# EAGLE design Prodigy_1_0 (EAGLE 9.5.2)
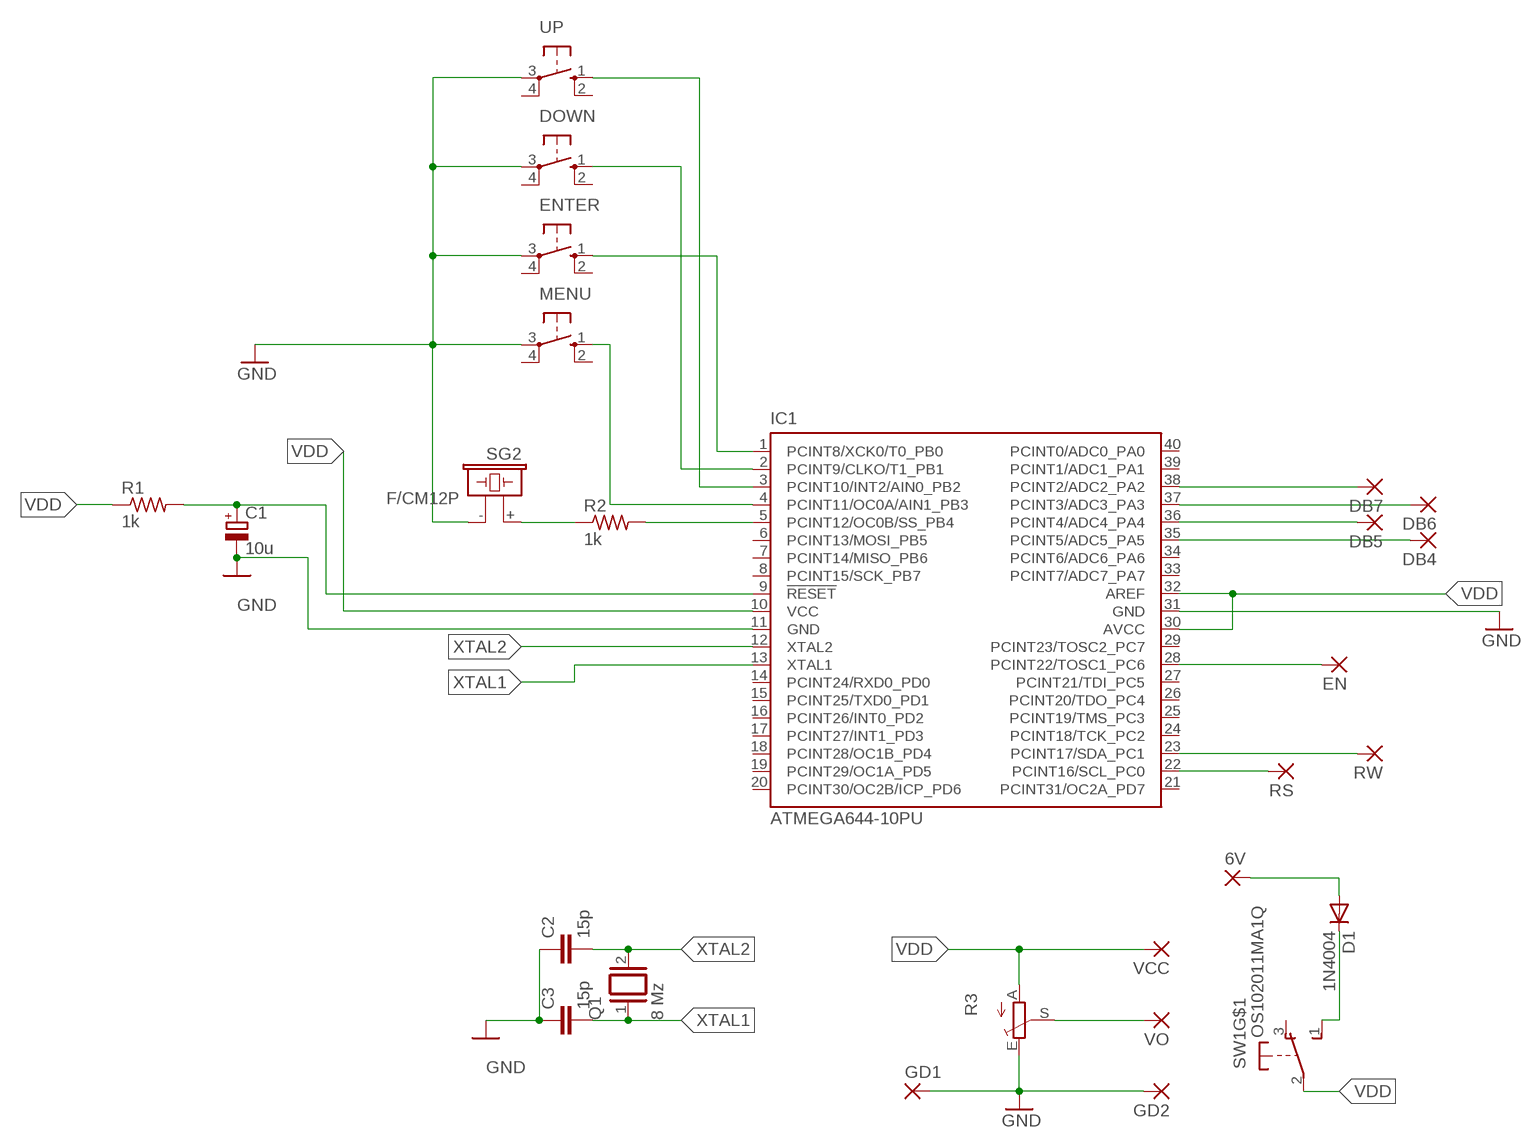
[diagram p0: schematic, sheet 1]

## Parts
6V  3,17/1,1  [3,17/1,1]
C1  10u  CPOL-EUB45181B  [B45181B]
C2  15p  C5/5  [C5B5]
C3  15p  C5/5  [C5B5]
D1  1N4004  [DO41-10]
DB4  3,17/1,1  [3,17/1,1]
DB5  3,17/1,1  [3,17/1,1]
DB6  3,17/1,1  [3,17/1,1]
DB7  3,17/1,1  [3,17/1,1]
DOWN  10-XX  [B3F-10XX]
EN  3,17/1,1  [3,17/1,1]
ENTER  10-XX  [B3F-10XX]
GD1  3,17/1,1  [3,17/1,1]
GD2  3,17/1,1  [3,17/1,1]
IC1  ATMEGA644-10PU  [DIL40]
MENU  10-XX  [B3F-10XX]
Q1  8 Mz  XTAL/S  [QS]
R1  1k  R-US_0204/7  [0204/7]
R2  1k  R-US_0204/7  [0204/7]
R3  TRIM_EU-LI10  [LI10]
RS  3,17/1,1  [3,17/1,1]
RW  3,17/1,1  [3,17/1,1]
SG2  F/CM12P  [F/CM12P]
SW1  OS102011MA1Q  [OS102011MA1Q]
UP  10-XX  [B3F-10XX]
VCC  3,17/1,1  [3,17/1,1]
VO  3,17/1,1  [3,17/1,1]

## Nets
GND: C1.- C2.1 C3.1 DOWN.3(P) ENTER.3(P) GD1.1(P) GD2.1(P) IC1.11(GND) IC1.31(GND) MENU.3(P) R3.E SG2.- UP.3(P)
N$1: ENTER.1(S) IC1.1(PCINT8/XCK0/T0_PB0)
N$2: DOWN.1(S) IC1.2(PCINT9/CLKO/T1_PB1)
N$3: DB7.1(P) IC1.38(PCINT2/ADC2_PA2)
N$4: C1.+ IC1.9(!RESET) R1.2
N$5: IC1.3(PCINT10/INT2/AIN0_PB2) UP.1(S)
N$6: IC1.4(PCINT11/OC0A/AIN1_PB3) MENU.1(S)
N$7: R2.1 SG2.+
N$8: EN.1(P) IC1.28(PCINT22/TOSC1_PC6)
N$9: DB5.1(P) IC1.36(PCINT4/ADC4_PA4)
N$10: IC1.23(PCINT17/SDA_PC1) RW.1(P)
N$11: DB4.1(P) IC1.35(PCINT5/ADC5_PA5)
N$12: DB6.1(P) IC1.37(PCINT3/ADC3_PA3)
N$13: IC1.22(PCINT16/SCL_PC0) RS.1(P)
N$14: D1.C SW1.1(S)
N$15: R3.S VO.1(P)
N$16: 6V.1(P) D1.A
N$17: IC1.5(PCINT12/OC0B/SS_PB4) R2.2
VDD: IC1.10(VCC) IC1.30(AVCC) IC1.32(AREF) R1.1 R3.A SW1.2(P) VCC.1(P)
XTAL1: C3.2 IC1.13(XTAL1) Q1.1
XTAL2: C2.2 IC1.12(XTAL2) Q1.2
Unconnected: DOWN.2(S1) DOWN.4(P1) ENTER.2(S1) ENTER.4(P1) IC1.6(PCINT13/MOSI_PB5) IC1.7(PCINT14/MISO_PB6) IC1.8(PCINT15/SCK_PB7) IC1.14(PCINT24/RXD0_PD0) IC1.15(PCINT25/TXD0_PD1) IC1.16(PCINT26/INT0_PD2) IC1.17(PCINT27/INT1_PD3) IC1.18(PCINT28/OC1B_PD4) IC1.19(PCINT29/OC1A_PD5) IC1.20(PCINT30/OC2B/ICP_PD6) IC1.21(PCINT31/OC2A_PD7) IC1.24(PCINT18/TCK_PC2) IC1.25(PCINT19/TMS_PC3) IC1.26(PCINT20/TDO_PC4) IC1.27(PCINT21/TDI_PC5) IC1.29(PCINT23/TOSC2_PC7) IC1.33(PCINT7/ADC7_PA7) IC1.34(PCINT6/ADC6_PA6) IC1.39(PCINT1/ADC1_PA1) IC1.40(PCINT0/ADC0_PA0) MENU.2(S1) MENU.4(P1) SW1.3(O) SW1.MT1(MT) SW1.MT2(MT) UP.2(S1) UP.4(P1)

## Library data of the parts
6V DB4-DB7 EN GD1 GD2 RS RW VCC VO = wirepad:3,17/1,1: THROUGH-HOLE PAD; OC_NEWARK: unknown
C1 = rcl:CPOL-EU: POLARIZED CAPACITOR, European symbol; SPICEPREFIX: C
C2 C3 = capacitor-wima:C: CAPACITOR; OC_NEWARK: unknown
D1 = adafruit:1N4004: DIODE; OC_NEWARK: unknown
DOWN ENTER MENU UP = switch-omron:10-XX: OMRON SWITCH; MF: OMRON ELECTRONIC COMPONENTS; MPN: B3F-1000; OC_FARNELL: 176432; OC_NEWARK: 36M3542
IC1 = atmel:ATMEGA644-*PU: 8-bit Microcontroller with 64K Bytes In-System Programmable Flash Auto generated by make-symbol-device-package-bsdl.ulp Rev. 34 Source: http://www.atmel.com/dyn/resources/prod_documents/doc2593.pdf; MPN: ATMEGA644V-10PU; OC_FARNELL: 1288342; OC_NEWARK: unknown
Q1 = special:XTAL/S: CRYSTAL
R1 R2 = adafruit:R-US_: RESISTOR, American symbol
R3 = pot:TRIM_EU-: POTENTIOMETER
SG2 = buzzer:F/CM12P: BUZZER; OC_FARNELL: unknown; OC_NEWARK: unknown
SW1 = adafruit:OS102011MA1Q: OS10201MA1Q through-hole right angle switch http://www.ladyada.net/library/eagle

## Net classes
0 default: width 0.127 mm, drill 0.127 mm, clearance 0.127 mm

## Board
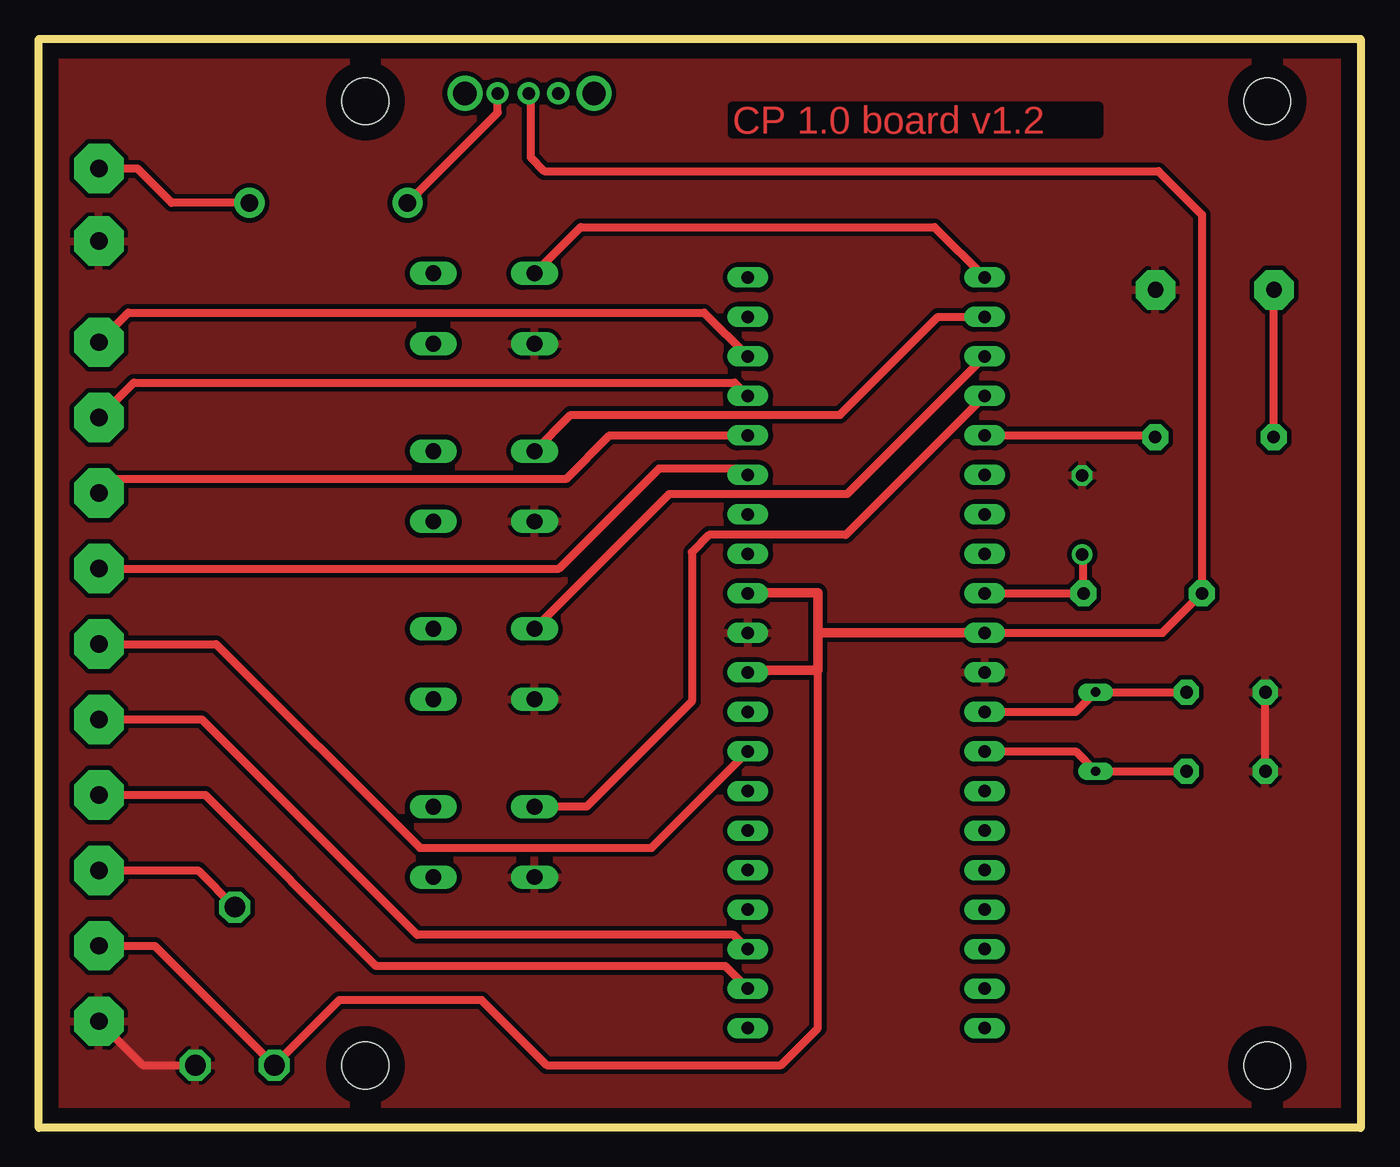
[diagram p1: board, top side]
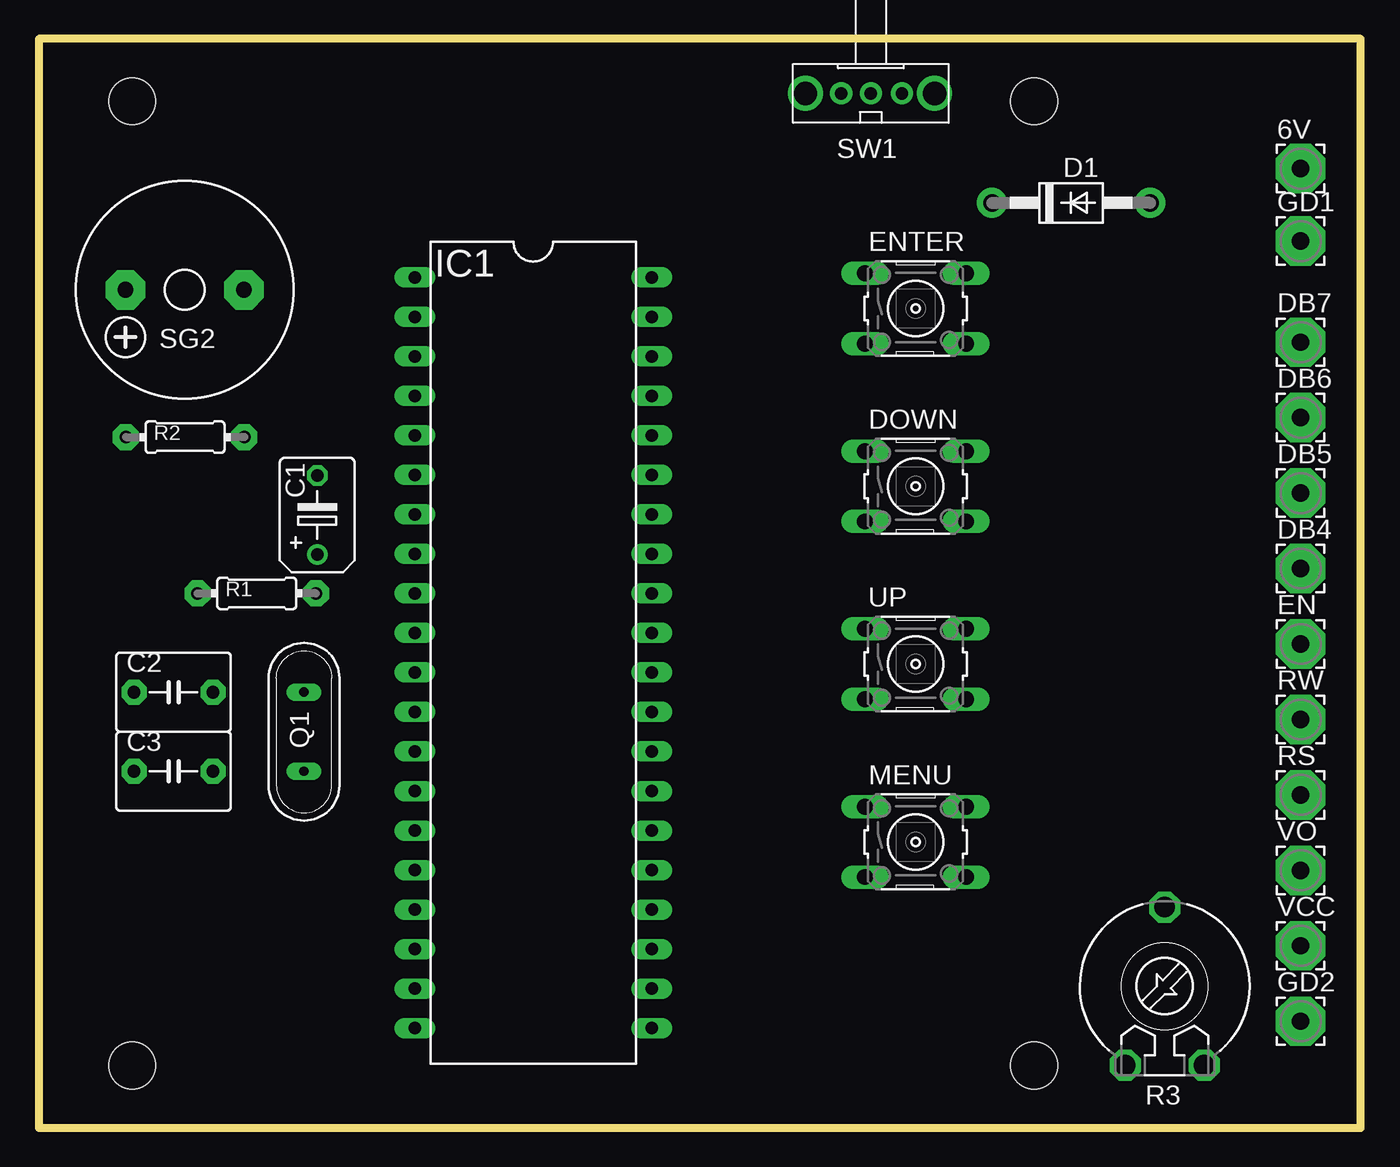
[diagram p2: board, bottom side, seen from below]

Size 85 x 70 mm. Coordinates in mm from the lower left corner, seen from the top.
Outline: 0,70 85,70 85,0 0,0 0,70
Copper layers (1*16): Top 0.035mm / dielectric 1.5mm / Bottom 0.035mm
Design rules "default *": minimum track width 6mil, minimum drill 0.35mm, track to track 12mil, track to pad 12mil, pad to pad 10mil, via to via 10mil, smd to smd 10mil, copper to edge 40mil, drill to drill 6mil, minimum pad ring 10mil, minimum via ring 8mil, stop-mask expansion 4mil, vias tented up to drill 0mil, thermal gap 10mil
Holes 3 mm at 21,4 79,4 79,66 21,66

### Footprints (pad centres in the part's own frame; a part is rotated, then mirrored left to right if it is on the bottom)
3,17/1,1 = drill 1.118 pad 3.175 octagon: 1 0,0
B45181B = drill 0.813: + -2.54,0 | drill 0.813 octagon: - 2.54,0
C5B5 = drill 0.813 pad 1.6 octagon: 1 -2.54,0; 2 2.54,0
DO41-10 = drill 1.118 pad 1.93: A 5.08,0; C -5.08,0
B3F-10XX = drill 1.016 long: 1 -3.251,2.261; 2 3.251,2.261; 3 -3.251,-2.261; 4 3.251,-2.261
DIL40 = drill 0.813 long: 1 -24.13,-7.62; 2 -21.59,-7.62; 3 -19.05,-7.62; 4 -16.51,-7.62; 5 -13.97,-7.62; 6 -11.43,-7.62; 7 -8.89,-7.62; 8 -6.35,-7.62; 9 -3.81,-7.62; 10 -1.27,-7.62; 11 1.27,-7.62; 12 3.81,-7.62; 13 6.35,-7.62; 14 8.89,-7.62; 15 11.43,-7.62; 16 13.97,-7.62; 17 16.51,-7.62; 18 19.05,-7.62; 19 21.59,-7.62; 20 24.13,-7.62; 21 24.13,7.62; 22 21.59,7.62; 23 19.05,7.62; 24 16.51,7.62; 25 13.97,7.62; 26 11.43,7.62; 27 8.89,7.62; 28 6.35,7.62; 29 3.81,7.62; 30 1.27,7.62; 31 -1.27,7.62; 32 -3.81,7.62; 33 -6.35,7.62; 34 -8.89,7.62; 35 -11.43,7.62; 36 -13.97,7.62; 37 -16.51,7.62; 38 -19.05,7.62; 39 -21.59,7.62; 40 -24.13,7.62
QS = drill 0.61 long: 1 -2.54,0; 2 2.54,0
0204/7 = drill 0.813 pad 1.676 octagon: 1 -3.81,0; 2 3.81,0
LI10 = drill 1.321 octagon: A -2.54,-5.08; E 2.54,-5.08; S 0,5.08
F/CM12P = drill 1.016 pad 2.54 octagon: + 3.81,0; - -3.81,0
OS102011MA1Q = drill 0.8 pad 1.422: 1 -2,0; 2 0,0; 3 1.9,0 | drill 1.5 pad 2.184: MT1 -4.1,0; MT2 4.2,0

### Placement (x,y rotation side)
6V  3.86,61.66 0 bottom
C1  67.1,39.4 90 bottom
C2  76.34,28 0 bottom
C3  76.34,22.92 0 bottom
D1  18.62,59.46 0 bottom
DB4  3.86,35.95 0 bottom
DB5  3.86,40.8 0 bottom
DB6  3.86,45.65 0 bottom
DB7  3.86,50.5 0 bottom
DOWN  28.62,41.24 0 bottom
EN  3.86,31.1 0 bottom
ENTER  28.62,52.67 0 bottom
GD1  3.86,57 0 bottom
GD2  3.86,6.85 0 bottom
IC1  53.21,30.54 270 bottom
MENU  28.62,18.38 0 bottom
Q1  67.95,25.46 90 bottom
R1  70.99,34.35 0 bottom
R2  75.6,44.4 0 bottom
R3  12.6,9.1 0 bottom
RS  3.86,21.4 0 bottom
RW  3.86,26.25 0 bottom
SG2  75.62,53.87 180 bottom
SW1  31.5,66.5 180 bottom
UP  28.62,29.81 0 bottom
VCC  3.86,11.7 0 bottom
VO  3.86,16.55 0 bottom

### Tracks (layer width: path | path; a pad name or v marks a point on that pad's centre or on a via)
GND
  Top 0.508: C3.1 C2.1 | GD2.1 6.69,4.02 R3.E
  pour Top: 0,0 85,0 85,70 0,70
N$1
  Top 0.508: IC1.1 57.6,57.9 34.84,57.9 ENTER.1
N$2
  Top 0.508: IC1.2 57.83,52.13 51.53,45.83 34.2,45.83 DOWN.1
N$3
  Top 0.508: IC1.38 42.78,52.4 5.76,52.4 DB7.1
N$4
  Top 0.508: C1.+ 67.18,36.78 R1.2 IC1.9
N$5
  Top 0.508: IC1.3 51.99,40.75 40.55,40.75 UP.1
N$6
  Top 0.508: IC1.4 51.89,38.11 43.11,38.11 42,37 42,27.41 35.23,20.64 MENU.1
N$7
  Top 0.508: R2.1 79.41,53.85 SG2.+
  Bottom 0.152: 79.41,53.85 SG2.+
N$8
  Top 0.508: EN.1 11.4,31.1 24.5,18 39.4,18 IC1.28
N$9
  Top 0.508: IC1.36 36.71,44.51 33.9,41.7 4.76,41.7 DB5.1
N$10
  Top 0.508: IC1.23 44.68,12.4 24.33,12.4 10.48,26.25 RW.1
N$11
  Top 0.508: IC1.35 45.19,42.37 39.87,42.37 33.45,35.95 DB4.1
N$12
  Top 0.508: IC1.37 44.74,47.9 6.11,47.9 DB6.1
N$13
  Top 0.508: IC1.22 44.14,10.4 21.7,10.4 10.7,21.4 RS.1
N$14
  Top 0.508: D1.C 29.5,65.26 SW1.1
N$15
  Top 0.508: R3.S 10.23,16.55 VO.1
N$16
  Top 0.508: 6V.1 6.34,61.66 8.54,59.46 D1.A
N$17
  Top 0.508: IC1.5 71.68,44.51 R2.2
  Top 0.61: 60.94,44.4 IC1.5
VDD
  Top 0.152: 60.74,31.9 IC1.10
  Top 0.508: IC1.10 72.26,31.81 R1.1 74.8,58.7 72,61.5 32.5,61.5 31.62,62.38 31.62,66.38 SW1.2 | 50.1,29.4 50.1,6.4 47.73,4.03 32.65,4.03 28.48,8.2 19.32,8.2 R3.A 7.46,11.7 VCC.1
  Top 0.61: 60.92,31.9 IC1.10 50.19,31.81 50.1,31.9 | IC1.30 45.72,29.4 50.1,29.4 50.1,31.9 | 50.1,31.9 50.1,34.4 45.64,34.4 IC1.32
XTAL1
  Top 0.508: IC1.13 66.68,24.19 Q1.1 C3.2
XTAL2
  Top 0.508: IC1.12 66.68,26.73 Q1.2 C2.2

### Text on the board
Top: CP 1.0 board v1.2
